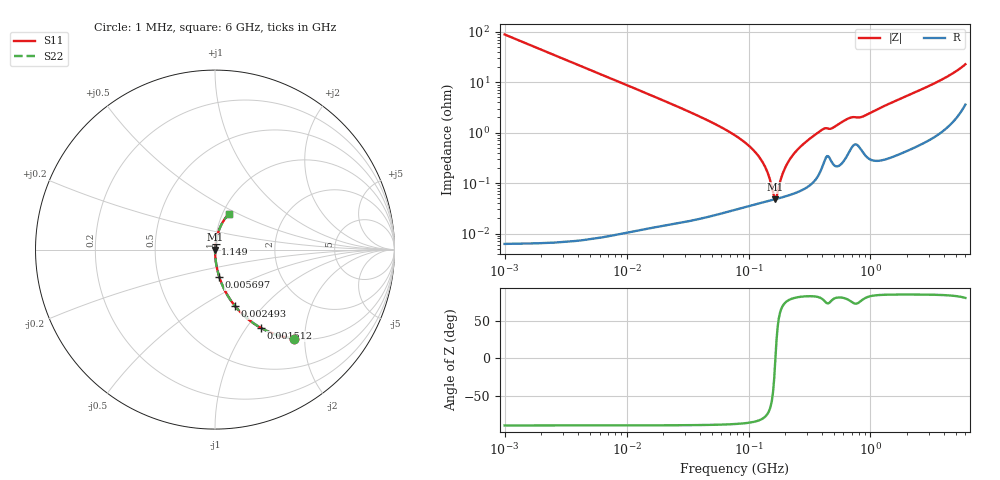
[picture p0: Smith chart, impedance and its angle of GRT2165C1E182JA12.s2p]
!Murata Part Number: GRT2165C1E182JA12
!These Parameters are Measured in Series Mode Connection
!Data Generated on Jun 19, 2026
!  o--ll--o
!Port1  Port2
!  o------o
!Operation Temp=25[degC], DC Bias Voltage=0[V]
!Freq. Start=1000[kHz] Stop=6[GHz] 401[Steps]
# Hz S RI R 50
!Freq.(Hz) S11(Real) S11(Imag) S21(Real) S21(Imag) S12(Real) S12(Imag) S22(Real) S22(Imag)
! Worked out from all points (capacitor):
!   401 points, 1 MHz to 6 GHz, reference 50 ohm
!   read as one part in series: C = 1.8 nF near 1.044 MHz
!   lowest |Z| = 48 mohm at 165.8 MHz (marker M1)
!   series resonance near 166.1 MHz, so ESL is about 510 pH
!   S11 on the Smith chart (normalised r, x): 1 MHz: 1.00, -1.77; 1.512 MHz: 1.00, -1.17; 2.493 MHz: 1.00, -0.71; 5.697 MHz: 1.00, -0.31; 1.149 GHz: 1.01, +0.06; 6 GHz: 1.07, +0.45
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1000000  0.4388 -0.4962  0.5612 0.4962  0.5612 0.4962  0.4388 -0.4962
1511688  0.2549 -0.4357  0.7451 0.4357  0.7451 0.4357  0.2549 -0.4357
2492906  0.1117 -0.3149  0.8883 0.3149  0.8883 0.3149  0.1117 -0.3149
4293785  0.0407 -0.1974  0.9593 0.1974  0.9593 0.1974  0.0407 -0.1974
5696791  0.0235 -0.1513  0.9765 0.1513  0.9765 0.1513  0.0235 -0.1513
1.843659e7  0.00237 -0.0472  0.9976 0.0472  0.9976 0.0472  0.00237 -0.0472
7.745967e7  0.000374 -0.00884  0.9996 0.00884  0.9996 0.00884  0.000374 -0.00884
1.027698e8  0.000383 -0.00524  0.9996 0.00524  0.9996 0.00524  0.000383 -0.00524
1.249896e8  0.000411 -0.00303  0.9996 0.00303  0.9996 0.00303  0.000411 -0.00303
1.424119e8  0.000438 -0.00162  0.9996 0.00162  0.9996 0.00162  0.000438 -0.00162
1.587717e8  0.000466 -0.000475  0.9995 0.000475  0.9995 0.000475  0.000466 -0.000475
1.658303e8  0.000479 -1.86e-05  0.9995 1.86e-05  0.9995 1.86e-05  0.000479 -1.86e-05
1.732027e8  0.000493 0.000438  0.9995 -0.000438  0.9995 -0.000438  0.000493 0.000438
1.930997e8  0.000533 0.00159  0.9995 -0.00159  0.9995 -0.00159  0.000533 0.00159
2.152823e8  0.000583 0.00276  0.9994 -0.00276  0.9994 -0.00276  0.000583 0.00276
2.561955e8  0.000694 0.00474  0.9993 -0.00474  0.9993 -0.00474  0.000694 0.00474
3.325952e8  0.00105 0.00817  0.9989 -0.00817  0.9989 -0.00817  0.00105 0.00817
4.133993e8  0.00264 0.0116  0.9974 -0.0116  0.9974 -0.0116  0.00264 0.0116
1.148954e9  0.0036 0.0291  0.9964 -0.0291  0.9964 -0.0291  0.0036 0.0291
1.428092e9  0.0045 0.0372  0.9955 -0.0372  0.9955 -0.0372  0.0045 0.0372
3.5601e9  0.019 0.0993  0.981 -0.0993  0.981 -0.0993  0.019 0.0993
6e9  0.0781 0.1998  0.9219 -0.1998  0.9219 -0.1998  0.0781 0.1998
